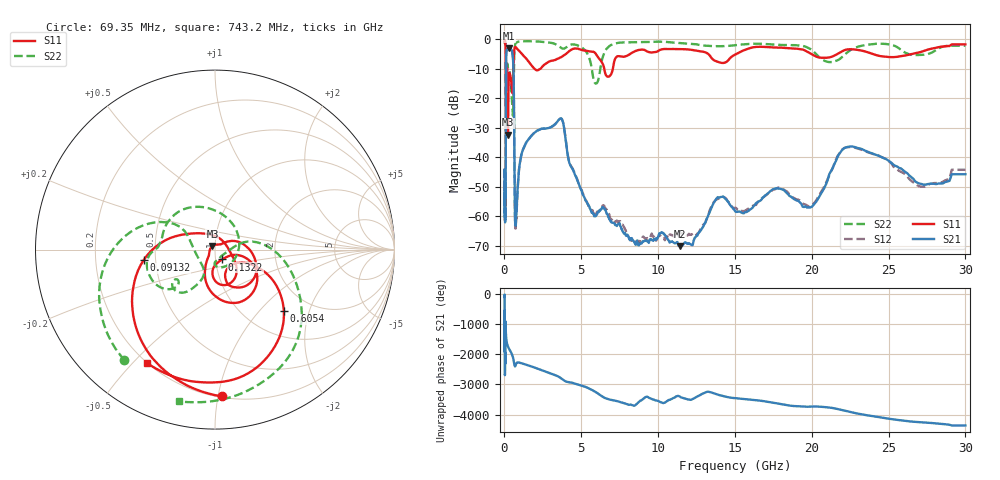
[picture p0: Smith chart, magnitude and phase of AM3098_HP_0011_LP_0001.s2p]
! Date/Time: Thu, Feb 28, 2019 8:33 AM
! Network Analyzer: Agilent Technologies E8364B Rev: A.07.50.67
! Sweep from 0.010 to 30.000 GHz, 1601 Points, Sweep Type: LOG
! Power Supply: 5.023 V, 0.002 A
# Hz S DB R 50
!freq MagS11 AngS11 MagS21 AngS21 MagS12 AngS12 MagS22 AngS22
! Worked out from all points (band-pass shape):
!   1601 points, 10 MHz to 30 GHz, reference 50 ohm
!   highest |S21| = -3.00 dB at 266.5 MHz (marker M1); lowest = -70.1 dB at 11.42 GHz (marker M2)
!   |S21| within 3 dB of the highest: 107.7 MHz to 546.2 MHz (438.5 MHz wide, 134 % of centre)
!   lowest |S11| = -32.3 dB at 228.2 MHz (marker M3), VSWR 1.05, Z = 48.5 + j1.91 ohm
!   |S11| at or under -10 dB: 175.5 MHz to 571.2 MHz (395.6 MHz wide, 106 % of centre); 1.966 GHz to 2.332 GHz (366 MHz wide, 17 % of centre); 6.497 GHz to 7.052 GHz (555.2 MHz wide, 8.2 % of centre)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
!   |S22| runs from -25.9 to -0.5 dB; largest |S21 - S12| = 0.011
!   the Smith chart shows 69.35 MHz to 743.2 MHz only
!   S11 on the Smith chart (normalised r, x): 69.35 MHz: 0.21, -1.03; 91.32 MHz: 0.43, -0.06; 132.2 MHz: 1.08, -0.12; 605.4 MHz: 1.47, -1.38; 743.2 MHz: 0.20, -0.55
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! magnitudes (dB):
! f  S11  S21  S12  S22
! 10 MHz  -0.4  -45.0  -44.0  -0.5
! 38.04 MHz  -0.5  -61.8  -60.5  -0.8
! 69.35 MHz  -1.7  -51.3  -54.4  -2.0
! 91.32 MHz  -7.9  -19.9  -19.8  -9.4
! 132.2 MHz  -23.4  -4.0  -3.9  -11.4
! 144.7 MHz  -14.3  -3.6  -3.6  -10.4
! 187.7 MHz  -11.6  -3.4  -3.4  -8.3
! 228.2 MHz  -32.3  -3.1  -3.1  -9.9
! 266.5 MHz  -15.1  -3.0  -3.0  -10.4
! 550.5 MHz  -13.5  -6.3  -6.2  -25.9
! 605.4 MHz  -5.8  -15.5  -15.4  -11.4
! 679.2 MHz  -2.6  -58.4  -58.5  -2.3
! 743.2 MHz  -2.7  -62.6  -62.5  -1.2
! 1.034 GHz  -4.4  -40.9  -40.8  -0.7
! 2.084 GHz  -10.5  -31.1  -31.1  -0.7
! 3.704 GHz  -6.0  -26.8  -26.9  -2.9
! 5.959 GHz  -5.0  -59.6  -59.3  -15.0
! 7.926 GHz  -5.7  -66.6  -65.4  -1.0
! 11.42 GHz  -3.3  -70.1  -65.7  -1.3
! 19.9 GHz  -4.8  -57.0  -56.8  -3.2
! 22.56 GHz  -3.3  -36.3  -36.5  -3.5
! 30 GHz  -1.7  -45.7  -44.2  -2.1
